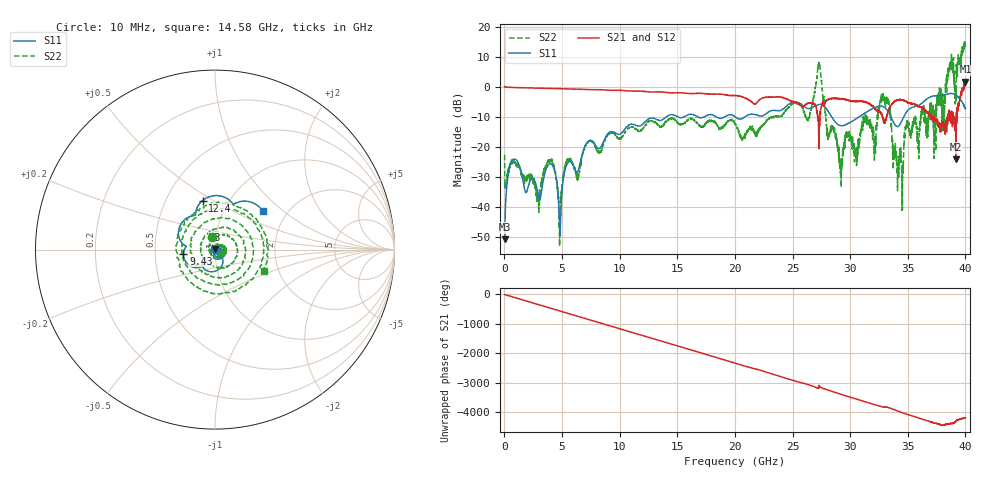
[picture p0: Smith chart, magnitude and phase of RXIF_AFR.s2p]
!Keysight Technologies,N5245B,MY58422297,A.13.80.12
!Automatic Fixture Removal (AFR)
!Date: Tuesday, April 21, 2020, 02:01:45
!S2P File: Measurements: S11,S21,S12,S22:
# MHz S  RI  R 50
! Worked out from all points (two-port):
!   4000 points, 10 MHz to 40 GHz, reference 50 ohm
!   highest |S21| = 1.67 dB at 40 GHz (marker M1); lowest = -24.2 dB at 39.19 GHz (marker M2)
!   |S21| within 3 dB of the highest: start of sweep to 10.43 GHz; 39.83061 GHz to end of sweep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
!   lowest |S11| = -50.7 dB at 10 MHz (marker M3), VSWR 1.01, Z = 50 + j0.289 ohm
!   |S11| at or under -10 dB: start of sweep to 14.05 GHz; 28.39 GHz to 30.8 GHz (2.414 GHz wide, 8.16 % of centre); 33.52 GHz to 34.65 GHz (1.128 GHz wide, 3.31 % of centre)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
!   |S22| runs from -53.0 to 15.4 dB; largest |S21 - S12| = 1.4e-15
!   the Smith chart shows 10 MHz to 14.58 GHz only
!   S11 on the Smith chart (normalised r, x): 10 MHz: 1.00, +0.01; 9.43 GHz: 0.70, -0.03; 12.4 GHz: 0.76, +0.45; 14.58 GHz: 1.51, +0.73
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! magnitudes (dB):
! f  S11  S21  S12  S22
! 10 MHz  -50.7  0.0  0.0  -22.6
! 770 MHz  -24.3  -0.3  -0.3  -24.4
! 2.91 GHz  -35.7  -0.5  -0.5  -37.6
! 4.1 GHz  -25.9  -0.6  -0.6  -24.1
! 4.81 GHz  -49.7  -0.7  -0.7  -43.2
! 5.41 GHz  -25.9  -0.8  -0.8  -24.5
! 6.68 GHz  -23.5  -0.9  -0.9  -24.0
! 9.43 GHz  -15.0  -1.2  -1.2  -15.4
! 12.4 GHz  -11.0  -1.7  -1.7  -12.0
! 13.34 GHz  -11.1  -1.7  -1.7  -12.9
! 14.58 GHz  -9.3  -2.1  -2.1  -10.5
! 20.01 GHz  -10.0  -2.9  -2.9  -12.3
! 26.67 GHz  -7.0  -5.5  -5.5  -6.8
! 27.34 GHz  -5.9  -13.1  -13.1  7.6
! 28.05 GHz  -7.9  -4.4  -4.4  -16.1
! 29.2 GHz  -13.0  -4.1  -4.1  -24.5
! 33.34 GHz  -8.6  -7.7  -7.7  -4.2
! 33.93 GHz  -12.9  -4.7  -4.7  -22.0
! 34.41 GHz  -11.9  -4.4  -4.4  -22.6
! 34.92 GHz  -8.3  -5.1  -5.1  -12.3
! 39.19 GHz  -2.8  -24.2  -24.2  -3.6
! 40 GHz  -7.3  1.7  1.7  14.0
